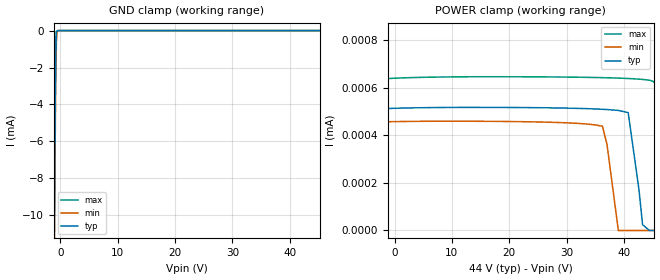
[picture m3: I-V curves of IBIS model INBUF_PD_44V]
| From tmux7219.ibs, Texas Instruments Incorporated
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| Model6
[Model]   INBUF_PD_44V
Model_type   Input
Vinl = 0.8
Vinh = 1.3
|   typ   min   max
C_comp   1.85pF   1.7pF   2.1pF
[Voltage Range]   44   39.6   48.4
[Temperature Range]   27   130   -40
[Power Clamp Reference]   44   39.6   48.4
[GND Clamp Reference]   0   0   0
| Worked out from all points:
|   GND clamp passes 1 mA (typ) near -0.78 V on its own axis
[GND Clamp]
|   Voltage   I(typ)   I(min)   I(max)
-44V      -2.328A    -2.326A    -2.332A
-1.1V     -12.66mA   -14.24mA   -11.59mA
-968mV    -6.594mA   -8.321mA   -5.409mA
-836mV    -1.77mA    -3.378mA   -813.6uA
-704mV    -86.03uA   -612uA     -49.19uA
-572mV    -14.17uA   -32.03uA   -21.99uA
-440mV    -2.586uA   -3.661uA   -4.159uA
88V       0A         0A         0A
[POWER Clamp]
|   Voltage   I(typ)   I(min)   I(max)
-44V      1.16mA     539.3uA    2.119mA
-15.22V   184.6uA    4.744uA    640.7uA
-11V      14.89uA    444.3nA    314.4uA
-10.6V    2.402uA    445.3nA    283.5uA
-10.34V   492.9nA    446nA      262.9uA
-6.776V   503.1nA    452.2nA    913.1nA
-6.644V   503.5nA    452.4nA    616.3nA
36.26V    508.7nA    437.4nA    641.5nA
40.74V    494.7nA    0A         637.9nA
44.44V    0A         0A         630.7nA
48.14V    0A         0A         0A
88V       0A         0A         0A
